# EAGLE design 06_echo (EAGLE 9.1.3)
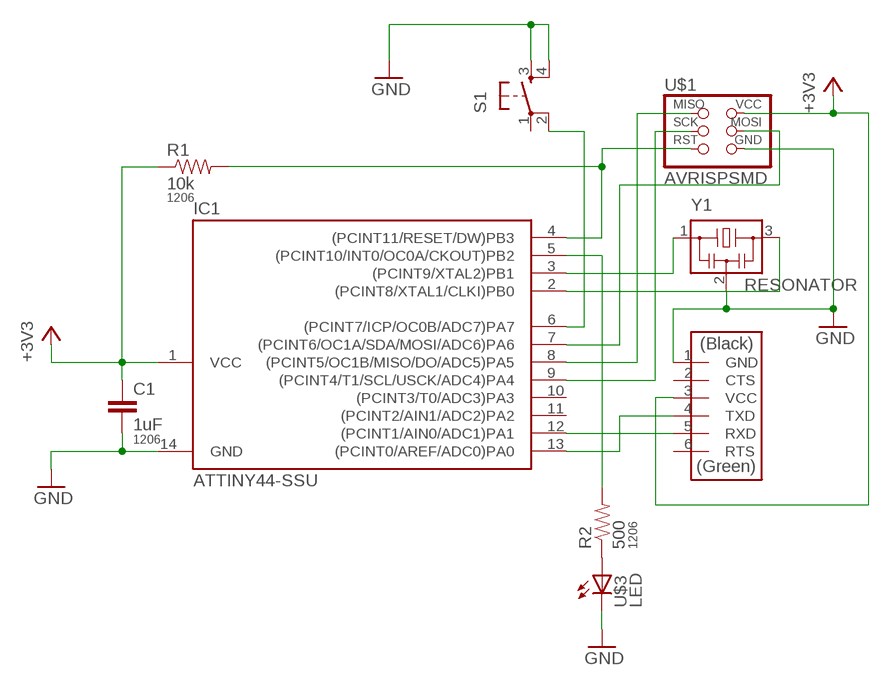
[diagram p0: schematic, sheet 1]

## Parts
C1  1uF  CAP1206  [1206]
IC1  ATTINY44-SSU  [SOIC14]
R1  10k  RESISTOR1206  [1206]
R2  500  RESISTOR1206  [1206]
S1  6MM_SWITCH6MM_SWITCH  [6MM_SWITCH]
U$1  AVRISPSMD  [2X03SMD]
U$2  FTDI-SMD-HEADER  [1X06SMD]
U$3  LED  [LED1206]
Y1  RESONATOR  [RES_EFOBM]

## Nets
+3V3: C1.1 IC1.1(VCC) R1.1 U$1.2(VCC) U$2.3(VCC)
GND: C1.2 IC1.14(GND) S1.3(S) S1.4(S1) U$1.6(GND) U$2.1(GND) U$3.2(C) Y1.2
N$1: IC1.13((PCINT0/AREF/ADC0)PA0) U$2.4(TXD)
N$2: IC1.4((PCINT11/RESET/DW)PB3) R1.2 U$1.5(RST)
N$3: IC1.12((PCINT1/AIN0/ADC1)PA1) U$2.5(RXD)
N$4: IC1.3((PCINT9/XTAL2)PB1) Y1.1
N$5: IC1.2((PCINT8/XTAL1/CLKI)PB0) Y1.3
N$6: IC1.9((PCINT4/T1/SCL/USCK/ADC4)PA4) U$1.3(SCK)
N$7: IC1.7((PCINT6/OC1A/SDA/MOSI/ADC6)PA6) U$1.4(MOSI)
N$8: IC1.8((PCINT5/OC1B/MISO/DO/ADC5)PA5) U$1.1(MISO)
N$9: IC1.5((PCINT10/INT0/OC0A/CKOUT)PB2) R2.2
N$10: R2.1 U$3.1(A)
N$11: IC1.6((PCINT7/ICP/OC0B/ADC7)PA7) S1.2(P1)
Unconnected: IC1.10((PCINT3/T0/ADC3)PA3) IC1.11((PCINT2/AIN1/ADC2)PA2) S1.1(P) U$2.2(CTS) U$2.6(RTS)

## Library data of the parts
C1 = passives:CAP: Capacitor; PACKAGE: 1206
IC1 = fab:ATTINY44
R1 R2 = passives:RESISTOR: Resistor; PACKAGE: 1206
S1 = fab:6MM_SWITCH: OMRON SWITCH
U$1 = fab:AVRISP
U$2 = fab:FTDI-SMD-HEADER
U$3 = fab:LED: LED
Y1 = passives:RESONATOR

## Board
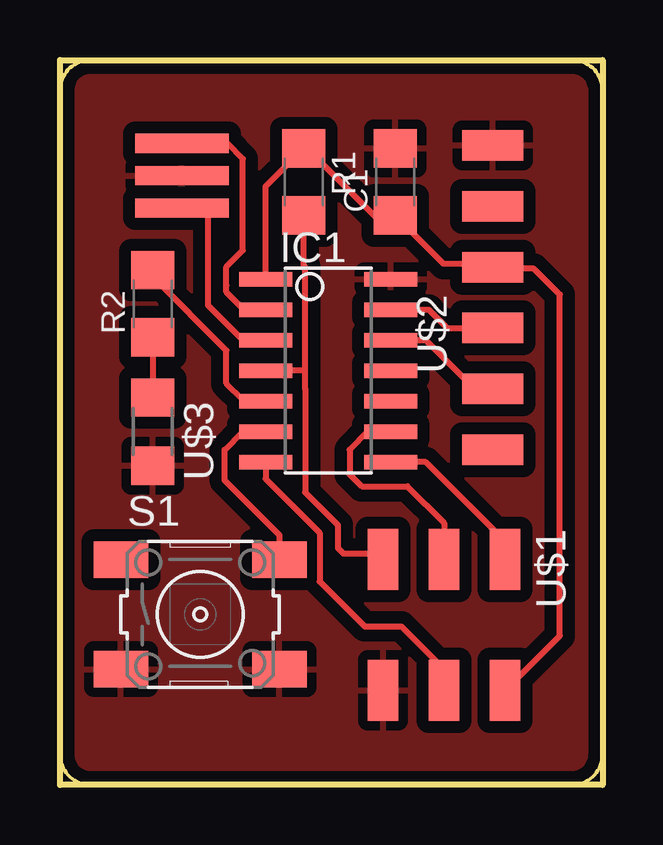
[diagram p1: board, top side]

Size 22.61 x 30.23 mm. Coordinates in mm from the lower left corner, seen from the top.
Outline: 21.34,30.23 1.27,30.23 arc90 0,28.96 0,1.27 arc90 1.27,0 21.34,0 arc90 22.61,1.27 22.61,28.96 arc90 21.34,30.23
Copper layers (1*16): Top 0.035mm / dielectric 1.5mm / Bottom 0.035mm
Design rules "fabcity-designrules": minimum track width 10mil, minimum drill 32mil, track to track 16mil, track to pad 16mil, pad to pad 16mil, via to via 16mil, smd to smd 6mil, copper to edge 16mil, drill to drill 16mil, minimum pad ring 10mil, minimum via ring 8mil, stop-mask expansion 4mil, vias tented up to drill 0mil, thermal gap 16mil
Milling: area 0,0 to 22.6,30.2

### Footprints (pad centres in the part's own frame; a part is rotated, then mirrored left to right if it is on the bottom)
1206 = smd 1.6 x 1.8: 1 -1.4,0; 2 1.4,0
SOIC14 = smd 0.61 x 2.21: 1 -3.81,-2.603; 2 -2.54,-2.603; 3 -1.27,-2.603; 4 0,-2.603; 5 1.27,-2.603; 6 2.54,-2.603; 7 3.81,-2.603; 8 3.81,2.603; 9 2.54,2.603; 10 1.27,2.603; 11 0,2.603; 12 -1.27,2.603; 13 -2.54,2.603; 14 -3.81,2.603
6MM_SWITCH = smd 2.286 x 1.524: 1 -3.302,2.286; 2 3.302,2.286; 3 -3.302,-2.286; 4 3.302,-2.286
2X03SMD = smd 2.54 x 1.27: 1 -2.54,2.54; 2 2.92,2.54; 3 -2.54,0; 4 2.92,0; 5 -2.54,-2.54; 6 2.92,-2.54
1X06SMD = smd 2.54 x 1.27: 1 0,6.35; 2 0,3.81; 3 0,1.27; 4 0,-1.27; 5 0,-3.81; 6 0,-6.35
LED1206 = smd 1.6 x 1.803: 1 -1.422,0; 2 1.422,0
RES_EFOBM = smd 0.8 x 3.9: 1 -1.35,0; 2 0,0; 3 1.35,0

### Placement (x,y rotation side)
C1  13.97,25.15 90 top
IC1  11.18,17.27 270 top
R1  10.16,25.15 270 top
R2  3.86,20.07 90 top
S1  5.84,7.11 0 top
U$1  16,6.86 270 top
U$2  18.03,20.32 0 top
U$3  3.86,14.73 270 top
Y1  5.08,25.4 90 top

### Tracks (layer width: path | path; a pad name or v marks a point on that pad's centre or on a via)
+3V3
  Top 0.254: U$1.2 20.83,6.22 20.83,20.45 19.75,21.53 18.1,21.53 U$2.3 17.91,21.72 16,21.72 C1.1 13.33,23.75 13.21,23.62 10.28,26.55 R1.1 8.57,24.96 IC1.1
GND
  pour Top (isolate 0.508): 23.62,32.51 23.62,-1.02 -1.78,-1.02 -1.78,32.51
N$1
  Top 0.254: IC1.13 15.37,19.81 16.13,19.05 U$2.4
N$2
  Top 0.254: U$1.5 13.46,9.65 11.81,9.65 11.58,9.88 11.58,10.83 10.21,12.2 10.21,16.53 10.21,17.27 | 10.21,17.27 10.21,21.61 10.16,21.66 R1.2 | 10.21,17.27 IC1.4
N$3
  Top 0.254: U$2.5 17.27,16.51 15.24,18.54 IC1.12
N$4
  Top 0.254: Y1.1 5.16,24.13 5.84,24.13 6.17,23.8 6.17,19.99 7.62,18.54 IC1.3
N$5
  Top 0.254: IC1.2 7.62,19.81 7.62,19.87 6.93,20.56 6.93,20.83 6.93,21.61 7.62,22.29 7.62,26.09 6.96,26.75 Y1.3
N$6
  Top 0.254: IC1.9 12.83,14.73 12.07,13.97 12.07,12.95 12.57,12.45 14.48,12.45 16,10.92 U$1.3
N$7
  Top 0.254: U$1.4 16,4.83 14.22,6.6 12.7,6.6 10.82,8.48 10.82,10.52 8.57,12.76 IC1.7
N$8
  Top 0.254: IC1.8 15.24,13.46 18.54,10.16 U$1.1
N$9
  Top 0.254: IC1.5 7.62,16 7.62,16.06 6.93,16.75 6.93,18.12 3.86,21.19 R2.2
N$10
  Top 0.254: R2.1 U$3.1
N$11
  Top 0.254: S1.2 9.14,10.41 6.86,12.7 6.86,13.97 7.62,14.73 IC1.6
